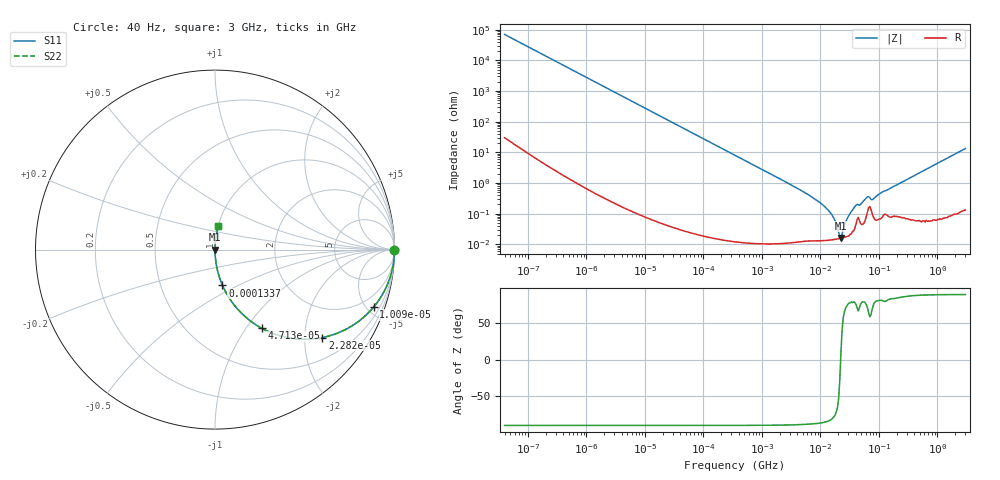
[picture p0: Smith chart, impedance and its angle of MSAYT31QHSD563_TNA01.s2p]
! MSAYT31QHSD563_TNA01  S-PARAMETER MODEL  ( General Type )
! Model Generated by TAIYO YUDEN Corporation (http://www.ty-top.com)
! Version 2.0
! TAIYO YUDEN Control No. 031016
! Copyright(c) 2003 TAIYO YUDEN CO.,LTD. All Rights Reserved.
! Product Description (link to TY-COMPAS)
! https://ds.yuden.co.jp/TYCOMPAS/or/detail?pn=MSAYT31QHSD563KTNA01&u=M
! Products Name : Multilayer Ceramic Capacitors
! Characteristics :
!  Capacitance : 0.056 uF , Rated Voltage : 25V
!  Case Size : 3.2 x 1.6 / 0.126 x 0.063 [mm/inch] , Thickness : 1.15 / 0.045 [mm/inch]
!  (Conditions: Temperature = 25 degC , DC Bias Current/Voltage = 0A / 0V)
! External Node Assignments :
!  1  o---| |---o  2
! GND o---------o GND
! Frequency Range : 40Hz  -  3GHz  [ 401 STEP ]
# MHz S RI R 50
! Freq[MHz].  S11 Real  S11 Imag  S21 Real  S21 Imag  S12 Real  S12 Imag  S22 Real  S22 Imag
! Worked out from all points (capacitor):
!   401 points, 40 Hz to 3 GHz, reference 50 ohm
!   read as one part in series: C = 57.1 nF near 44 Hz
!   lowest |Z| = 16.2 mohm at 22.43 MHz (marker M1)
!   series resonance near 22.15 MHz, so ESL is about 900 pH
!   S11 on the Smith chart (normalised r, x): 40 Hz: open; 10.09 kHz: 1.00, -5.52; 22.82 kHz: 1.00, -2.44; 47.13 kHz: 1.00, -1.18; 133.7 kHz: 1.00, -0.42; 3 GHz: 1.00, +0.27
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4e-05  1 -0.00144  2.68e-06 0.00144  2.68e-06 0.00144  1 -0.00144
0.000834  0.9991 -0.0299  0.000902 0.0299  0.000902 0.0299  0.9991 -0.0299
0.0034  0.9853 -0.1202  0.0147 0.1202  0.0147 0.1202  0.9853 -0.1202
0.010091  0.884 -0.32  0.116 0.32  0.116 0.32  0.884 -0.32
0.017386  0.7198 -0.4489  0.2802 0.4489  0.2802 0.4489  0.7198 -0.4489
0.022821  0.5986 -0.49  0.4014 0.49  0.4014 0.49  0.5986 -0.49
0.047134  0.2592 -0.4379  0.7408 0.4379  0.7408 0.4379  0.2592 -0.4379
0.077606  0.1144 -0.318  0.8856 0.318  0.8856 0.318  0.1144 -0.318
0.133706  0.0418 -0.1997  0.9582 0.1997  0.9582 0.1997  0.0418 -0.1997
0.362475  0.00599 -0.0764  0.994 0.0764  0.994 0.0764  0.00599 -0.0764
7.222098  0.000141 -0.00344  0.9999 0.00344  0.9999 0.00344  0.000141 -0.00344
14.25536  0.000138 -0.00116  0.9999 0.00116  0.9999 0.00116  0.000138 -0.00116
17.08948  0.000144 -0.000673  0.9999 0.000673  0.9999 0.000673  0.000144 -0.000673
20.48705  0.000153 -0.000199  0.9998 0.000199  0.9998 0.000199  0.000153 -0.000199
22.43131  0.000159 3.09e-05  0.9998 -3.09e-05  0.9998 -3.09e-05  0.000159 3.09e-05
23.47158  0.000162 0.000143  0.9998 -0.000143  0.9998 -0.000143  0.000162 0.000143
29.4429  0.000184 0.000748  0.9998 -0.000748  0.9998 -0.000748  0.000184 0.000748
38.64618  0.000338 0.00165  0.9997 -0.00165  0.9997 -0.00165  0.000338 0.00165
60.81113  0.00082 0.00314  0.9992 -0.00314  0.9992 -0.00314  0.00082 0.00314
79.8195  0.000811 0.00289  0.9992 -0.00289  0.9992 -0.00289  0.000811 0.00289
150.5692  0.000825 0.00637  0.9992 -0.00637  0.9992 -0.00637  0.000825 0.00637
3000  0.0185 0.1299  0.9815 -0.1299  0.9815 -0.1299  0.0185 0.1299
